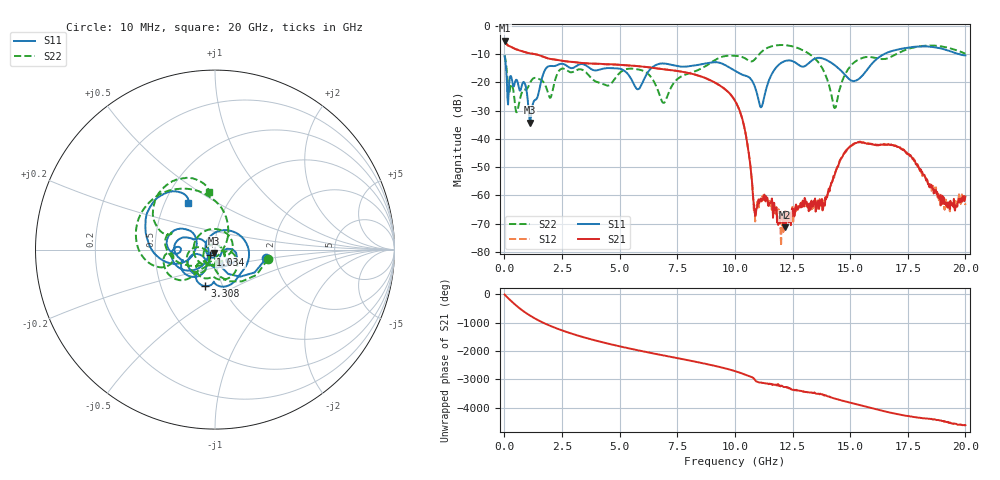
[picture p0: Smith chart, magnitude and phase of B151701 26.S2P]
!  2-Port S-parameters saved by WinCal
! VAR MeasName=S-Parameters (CALIBRATED_DATA) read from VNA (N5244A)
! VAR MeasDate=2015-12-24 19:11:09
! VAR NAME=B151701 26
! VAR FILENAME=B151701 26.S2P
! VAR DATE=2015-12-24 19:11:09
! VAR PHYS_PORTS=1,3
# Hz S DB R 50
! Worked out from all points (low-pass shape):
!   801 points, 10 MHz to 20 GHz, reference 50 ohm
!   highest |S21| = -5.17 dB at 10 MHz (marker M1); lowest = -71.4 dB at 12.15 GHz (marker M2)
!   |S21| within 3 dB of the highest: start of sweep to 476.4 MHz
!   lowest |S11| = -34.2 dB at 1.109 GHz (marker M3), VSWR 1.04, Z = 49.6 - j1.89 ohm
!   |S11| at or under -10 dB: start of sweep to 16.47 GHz; 19.72 GHz to end of sweep
!   |S22| runs from -30.6 to -6.8 dB; largest |S21 - S12| = 0.0019
!   S11 on the Smith chart (normalised r, x): 10 MHz: 1.79, -0.19; 1.034 GHz: 0.95, -0.05; 3.308 GHz: 0.82, -0.35; 20 GHz: 0.65, +0.37
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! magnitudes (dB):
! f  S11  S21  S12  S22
! 10 MHz  -10.8  -5.2  -5.1  -10.5
! 184.9 MHz  -23.5  -7.0  -7.0  -23.8
! 534.7 MHz  -19.1  -8.3  -8.3  -30.6
! 1.034 GHz  -28.0  -9.6  -9.6  -21.6
! 1.109 GHz  -34.2  -9.7  -9.7  -20.3
! 1.859 GHz  -14.6  -11.4  -11.4  -22.8
! 3.308 GHz  -13.5  -13.1  -13.1  -15.4
! 3.358 GHz  -13.5  -13.1  -13.1  -15.5
! 4.483 GHz  -14.9  -13.6  -13.6  -21.2
! 5.782 GHz  -22.5  -14.2  -14.2  -15.4
! 6.682 GHz  -13.5  -15.1  -15.1  -23.3
! 10.01 GHz  -15.9  -26.5  -26.5  -10.6
! 10.45 GHz  -17.6  -37.7  -37.6  -11.5
! 10.88 GHz  -21.8  -67.2  -69.3  -11.7
! 11.15 GHz  -28.7  -62.1  -62.2  -9.2
! 12.15 GHz  -12.5  -71.4  -69.5  -6.8
! 13.35 GHz  -12.1  -63.1  -64.8  -10.7
! 14.33 GHz  -13.9  -52.8  -52.9  -29.1
! 15.15 GHz  -19.6  -41.7  -42.0  -13.1
! 16.68 GHz  -9.2  -41.9  -41.9  -11.3
! 19.23 GHz  -8.6  -64.4  -62.7  -7.6
! 20 GHz  -10.5  -60.4  -63.4  -9.8
